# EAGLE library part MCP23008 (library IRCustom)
MCP23008 Inexpensive i2c i/o expander - 8 general purpose i/o pins with optional pullups
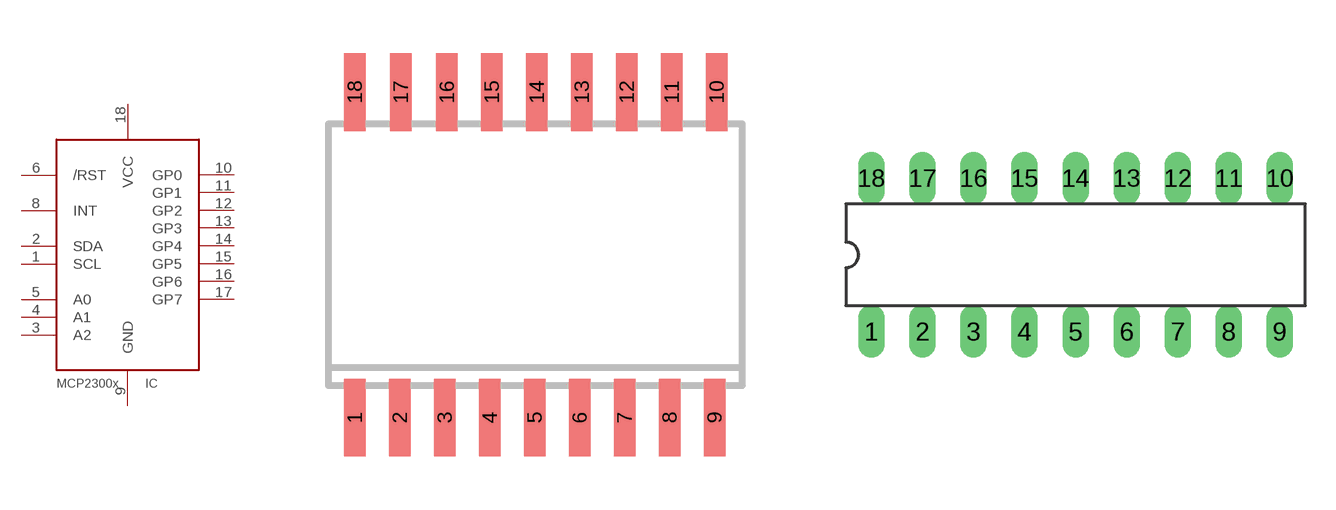
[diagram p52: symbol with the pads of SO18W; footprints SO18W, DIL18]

Designator prefix IC

## MCP23008/SO  [SO18W]
1  SCL
2  SDA
3  A2  in
4  A1  in
5  A0  in
6  /RST  in
8  INT  out
9  GND  pwr
10  GP0
11  GP1
12  GP2
13  GP3
14  GP4
15  GP5
16  GP6
17  GP7
18  VCC  pwr

## MCP23008/P  [DIL18]
Pads as for SO18W

## Footprint SO18W (pad centres in mm)
smd 0.6 x 2.2: 1 -4.445,-4.6; 2 -3.175,-4.6; 3 -1.905,-4.6; 4 -0.635,-4.6; 5 0.635,-4.6; 6 1.905,-4.6; 7 3.175,-4.6; 8 4.445,-4.6; 9 5.715,-4.6; 10 5.775,4.6; 11 4.505,4.6; 12 3.235,4.6; 13 1.965,4.6; 14 0.695,4.6; 15 -0.575,4.6; 16 -1.845,4.6; 17 -3.145,4.6; 18 -4.445,4.6

## Footprint DIL18 (pad centres in mm)
Dual In Line package type P
drill 0.813 long: 1 -10.16,-3.81; 2 -7.62,-3.81; 3 -5.08,-3.81; 4 -2.54,-3.81; 5 0,-3.81; 6 2.54,-3.81; 7 5.08,-3.81; 8 7.62,-3.81; 9 10.16,-3.81; 10 10.16,3.81; 11 7.62,3.81; 12 5.08,3.81; 13 2.54,3.81; 14 0,3.81; 15 -2.54,3.81; 16 -5.08,3.81; 17 -7.62,3.81; 18 -10.16,3.81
